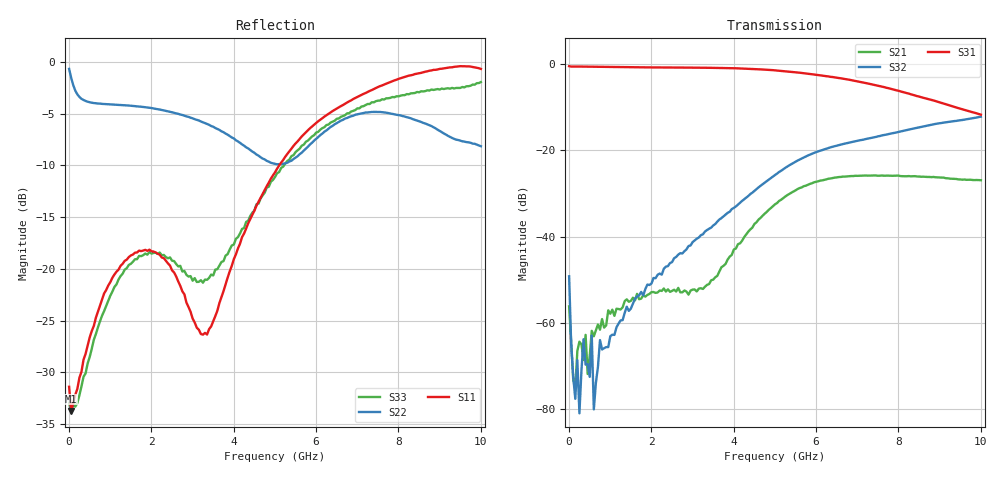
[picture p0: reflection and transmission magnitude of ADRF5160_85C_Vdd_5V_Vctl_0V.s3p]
! Device:  ADRF5160
! Description: Silicon SPDT Switch
! Frequency:  0.7 -  4 GHz
! Ports:
!	RFc	= Port 1
!	RF1	= Port 2
!  RF2  = Port 3
! Vdd:  5 Volt
! Control:  0 Volt
! Data:  Data was collected using a calibrated 4 port network analyzer and de-embedded using Agilent's AFR De-Embedding.
! Note:  Analog Devices supplies this data as a sample of measured data
!  for this product.  Your particular data for this product may vary.
!  Data was taken at 85 degrees C.
!S3P File: Measurements: <S11,S12,S13>,
!<S21,S22,S23>,
!<S31,S32,S33>:
# Hz S  dB  R 50
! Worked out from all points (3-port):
!   201 points, 10 MHz to 10 GHz, reference 50 ohm
!   strongest paths, dB at 10 MHz, 2.507 GHz, 5.005 GHz, 7.503 GHz, 10 GHz:
!     S31: -0.5, -0.8, -1.4, -5.0, -11.7
!     S32: -49.2, -45.9, -25.7, -16.7, -12.2
!     S21: -56.1, -52.5, -32.5, -25.9, -26.9
!   lowest |S11| = -33.8 dB at 59.95 MHz (marker M1), VSWR 1.04, Z = 52 - j0.556 ohm
!   |S11| at or under -10 dB: start of sweep to 5.105 GHz
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1e7  -31.41 3.9  -53.90 -54.1  -0.52 -0.5
     -56.11 -91.0  -0.65 -8.6  -59.34 165.5
     -0.46 -0.2  -49.15 3.7  -32.95 -12.8
5.995e7  -33.76 -15.1  -61.94 141.1  -0.54 -1.8
         -64.26 -127.1  -1.52 -45.2  -80.06 163.9
         -0.56 -1.7  -64.88 35.3  -33.98 -14.8
1.099e8  -32.98 -31.1  -74.89 -24.2  -0.54 -3.1
         -73.12 64.1  -2.23 -73.0  -71.53 9.5
         -0.54 -3.0  -72.51 -13.9  -32.96 -24.5
2.5975e8  -30.53 -50.3  -69.20 148.9  -0.57 -7.0
          -64.31 65.8  -3.37 -121.9  -69.63 -20.0
          -0.55 -7.0  -80.91 160.0  -32.22 -50.0
5.5945e8  -26.02 -74.8  -63.15 85.1  -0.57 -14.9
          -61.80 94.4  -3.93 -158.5  -67.80 -127.0
          -0.58 -15.1  -62.93 152.1  -27.73 -86.4
6.094e8  -25.52 -78.5  -62.59 79.7  -0.58 -16.3
         -63.05 90.1  -3.96 -161.9  -74.58 -155.5
         -0.59 -16.3  -80.00 -158.3  -26.86 -90.1
6.5935e8  -24.73 -79.4  -63.96 84.1  -0.58 -17.7
          -61.69 88.8  -3.98 -164.9  -74.49 -73.3
          -0.59 -17.6  -73.87 -114.0  -26.30 -96.0
5.005e9  -10.67 22.0  -32.51 100.6  -1.43 -139.4
         -32.48 100.9  -9.84 100.0  -25.65 113.0
         -1.43 -139.4  -25.69 113.1  -11.12 -131.5
7.5025e9  -2.41 -49.7  -25.85 -17.3  -4.99 143.7
          -25.86 -17.3  -4.83 73.4  -16.75 8.8
          -5.00 143.7  -16.72 8.9  -3.73 154.4
1e10  -0.66 -84.2  -26.90 -90.5  -11.69 85.7
      -26.89 -90.5  -8.14 -2.2  -12.15 -76.7
      -11.70 85.7  -12.16 -76.7  -1.93 77.2
